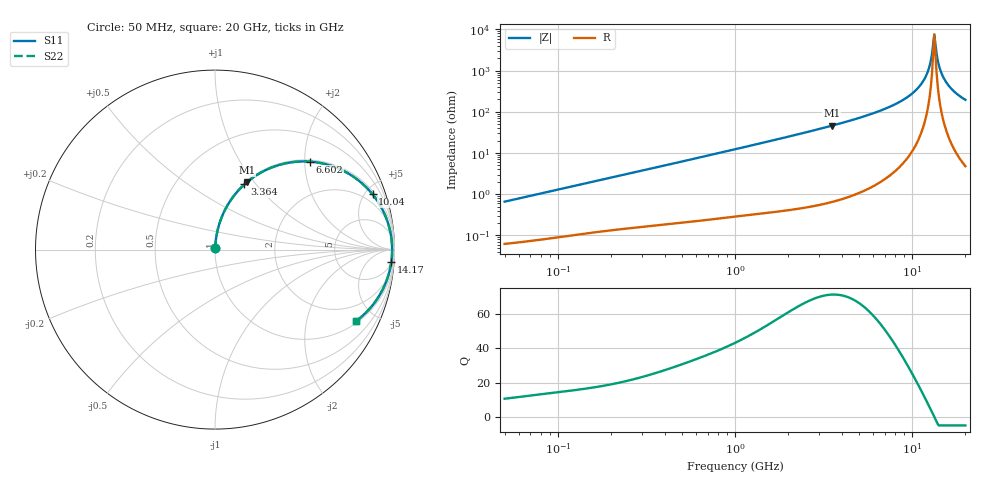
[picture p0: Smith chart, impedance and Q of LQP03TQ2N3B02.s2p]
!Murata Part Number: LQP03TQ2N3B02
!These Parameters are Measured in Series Mode Connection
!  o--[Z]--o
!Port1  Port2
!  o-------o
!Freq. Start=50[MHz] Stop=20[GHz], 401[Steps]
# Hz S RI R 50
!Freq.(Hz) S11(Real) S11(Imag) S21(Real) S21(Imag) S12(Real) S12(Imag) S22(Real) S22(Imag)
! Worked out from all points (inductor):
!   401 points, 50 MHz to 20 GHz, reference 50 ohm
!   read as one part in series: L = 2.08 nH near 51.52 MHz
!   highest Q = 71.2 at 3.519 GHz (marker M1), where L = 2.08 nH
!   self-resonance near 13.35 GHz
!   S11 on the Smith chart (normalised r, x): 50 MHz: 1.00, +0.01; 3.364 GHz: 1.01, +0.87; 6.602 GHz: 1.04, +2.12; 10.04 GHz: 1.23, +5.61; 14.17 GHz: 6, -26; 20 GHz: 1.10, -3.91
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5e7  0.000666 0.00657  0.9993 -0.00657  0.9993 -0.00657  0.000666 0.00657
1.364002e8  0.00138 0.0174  0.9986 -0.0174  0.9986 -0.0174  0.00138 0.0174
3.721004e8  0.0039 0.0461  0.9961 -0.0461  0.9961 -0.0461  0.0039 0.0461
1e9  0.0177 0.1209  0.9823 -0.1209  0.9823 -0.1209  0.0177 0.1209
2.728004e9  0.1109 0.3068  0.8891 -0.3068  0.8891 -0.3068  0.1109 0.3068
3.364474e9  0.1641 0.3634  0.8359 -0.3634  0.8359 -0.3634  0.1641 0.3634
3.519108e9  0.1783 0.3758  0.8217 -0.3758  0.8217 -0.3758  0.1783 0.3758
4.81993e9  0.3151 0.4572  0.6849 -0.4572  0.6849 -0.4572  0.3151 0.4572
6.601595e9  0.5298 0.49  0.4702 -0.49  0.4702 -0.49  0.5298 0.49
7.442007e9  0.6301 0.4723  0.3699 -0.4723  0.3699 -0.4723  0.6301 0.4723
1.004137e10  0.8779 0.308  0.1221 -0.308  0.1221 -0.308  0.8779 0.308
1.115139e10  0.9408 0.2071  0.0592 -0.2071  0.0592 -0.2071  0.9408 0.2071
1.201863e10  0.9707 0.1244  0.0293 -0.1244  0.0293 -0.1244  0.9707 0.1244
1.257102e10  0.9815 0.0721  0.0185 -0.0721  0.0185 -0.0721  0.9815 0.0721
1.314879e10  0.9865 0.0185  0.0135 -0.0185  0.0135 -0.0185  0.9865 0.0185
1.334722e10  0.9869 0.000564  0.0131 -0.000564  0.0131 -0.000564  0.9869 0.000564
1.375312e10  0.9857 -0.0353  0.0143 0.0353  0.0143 0.0353  0.9857 -0.0353
1.417136e10  0.9819 -0.071  0.0181 0.071  0.0181 0.071  0.9819 -0.071
1.482269e10  0.9715 -0.1235  0.0285 0.1235  0.0285 0.1235  0.9715 -0.1235
1.597544e10  0.9421 -0.2065  0.0579 0.2065  0.0579 0.2065  0.9421 -0.2065
1.774144e10  0.8796 -0.3081  0.1204 0.3081  0.1204 0.3081  0.8796 -0.3081
2e10  0.787 -0.3973  0.213 0.3973  0.213 0.3973  0.787 -0.3973
